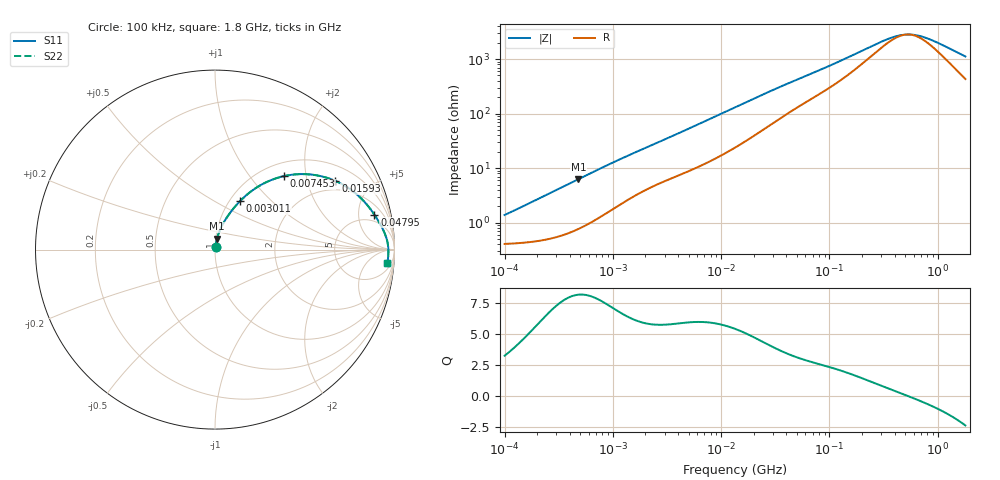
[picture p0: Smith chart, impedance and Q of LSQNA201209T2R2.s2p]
! LSQNA201209T2R2  S-PARAMETER MODEL  ( General Type )
! Model Generated by TAIYO YUDEN Corporation (http://www.ty-top.com)
! Version 2.0
! TAIYO YUDEN Control No. 100810NF25SB-FKC
! Copyright(c) 2007 TAIYO YUDEN CO.,LTD. All Rights Reserved.
! Product Description (link to TY-COMPAS)
! https://ds.yuden.co.jp/TYCOMPAS/or/detail?pn=LSQNA201209T2R2M&u=M
! Products Name : Inductors
! Characteristics :
!  Inductance : 2.2 uH , SRF(min) : 80 MHz , DC Resistance(max) : 0.507 Ohm
!  Rated Current : Saturation :440 mA , Temp Rise : 590 mA (40 degC)
!  Case Size : 2.0 x 1.25 / 0.079 x 0.049 [mm/inch] , Thickness : 0.9 / 0.035 [mm/inch]
!  (Conditions: Temperature = 25 degC , DC Bias Current/Voltage = 0A / 0V)
! External Node Assignments :
!  1  o---GGG---o  2
! GND o---------o GND
! Frequency Range : 0.1MHz  -  1800MHz  [ 402 STEP ]
# MHz S RI R 50
! Freq[MHz].  S11 Real  S11 Imag  S21 Real  S21 Imag  S12 Real  S12 Imag  S22 Real  S22 Imag
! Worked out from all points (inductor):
!   401 points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, 100 kHz to 1.8 GHz, reference 50 ohm
!   read as one part in series: L = 2.1 uH near 105 kHz
!   highest Q = 8.17 at 479.6 kHz (marker M1), where L = 2.07 uH
!   self-resonance near 524.8 MHz
!   S11 on the Smith chart (normalised r, x): 100 kHz: 1.01, +0.03; 3.011 MHz: 1.12, +0.66; 7.453 MHz: 1.25, +1.50; 15.93 MHz: 1.58, +3.00; 47.95 MHz: 3.43, +7.71; 1.8 GHz: 10, -21
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0.1  0.00423 0.0131  0.9958 -0.0131  0.9958 -0.0131  0.00423 0.0131
0.479561  0.0114 0.0612  0.9886 -0.0612  0.9886 -0.0612  0.0114 0.0612
0.516129  0.0125 0.0657  0.9875 -0.0657  0.9875 -0.0657  0.0125 0.0657
1.277529  0.0457 0.1459  0.9543 -0.1459  0.9543 -0.1459  0.0457 0.1459
2.66389  0.1197 0.2489  0.8803 -0.2489  0.8803 -0.2489  0.1197 0.2489
3.010975  0.1388 0.2695  0.8612 -0.2695  0.8612 -0.2695  0.1388 0.2695
4.679446  0.2336 0.3469  0.7664 -0.3469  0.7664 -0.3469  0.2336 0.3469
7.452807  0.3845 0.4095  0.6155 -0.4095  0.6155 -0.4095  0.3845 0.4095
9.999495  0.4982 0.4206  0.5018 -0.4206  0.5018 -0.4206  0.4982 0.4206
13.41641  0.6108 0.4039  0.3892 -0.4039  0.3892 -0.4039  0.6108 0.4039
15.92588  0.6705 0.3828  0.3295 -0.3828  0.3295 -0.3828  0.6705 0.3828
26.63823  0.8057 0.2936  0.1943 -0.2936  0.1943 -0.2936  0.8057 0.2936
47.95365  0.8879 0.1949  0.1121 -0.1949  0.1121 -0.1949  0.8879 0.1949
69.24595  0.9172 0.1474  0.0828 -0.1474  0.0828 -0.1474  0.9172 0.1474
147.9715  0.9516 0.0747  0.0484 -0.0747  0.0484 -0.0747  0.9516 0.0747
357.3983  0.9644 0.0191  0.0356 -0.0191  0.0356 -0.0191  0.9644 0.0191
424.248  0.9652 0.0105  0.0348 -0.0105  0.0348 -0.0105  0.9652 0.0105
491.4156  0.9657 0.00321  0.0343 -0.00321  0.0343 -0.00321  0.9657 0.00321
569.2172  0.9659 -0.00399  0.0341 0.00399  0.0341 0.00399  0.9659 -0.00399
659.3364  0.966 -0.0113  0.034 0.0113  0.034 0.0113  0.966 -0.0113
906.5744  0.9655 -0.0282  0.0345 0.0282  0.0345 0.0282  0.9655 -0.0282
1800  0.9604 -0.0768  0.0396 0.0768  0.0396 0.0768  0.9604 -0.0768
